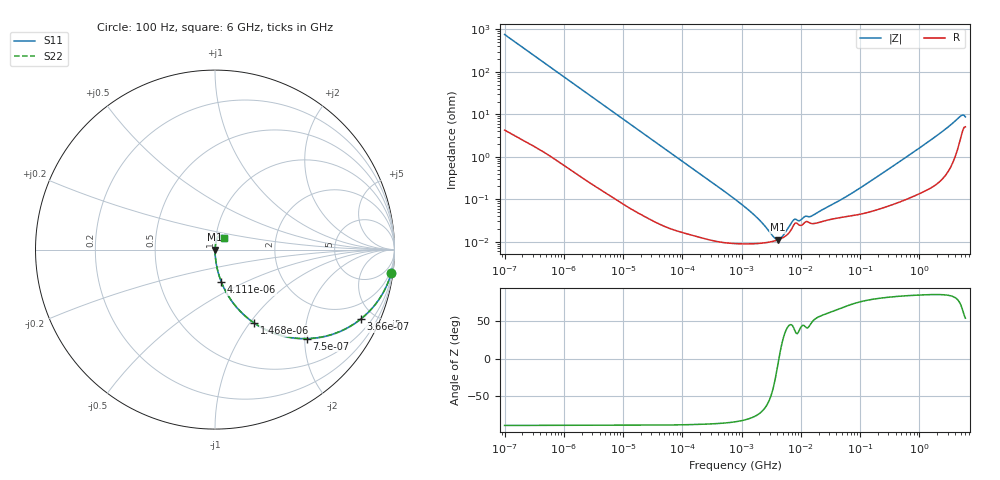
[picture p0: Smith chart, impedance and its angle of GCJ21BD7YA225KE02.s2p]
!Murata Part Number: GCJ21BD7YA225KE02
!These Parameters are Measured in Series Mode Connection
!Data Generated on Mar 13, 2026
!  o--ll--o
!Port1  Port2
!  o------o
!Operation Temp=25[degC], DC Bias Voltage=0[V]
!Freq. Start=100[Hz] Stop=6[GHz] 401[Steps]
# Hz S RI R 50
!Freq.(Hz) S11(Real) S11(Imag) S21(Real) S21(Imag) S12(Real) S12(Imag) S22(Real) S22(Imag)
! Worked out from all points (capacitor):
!   401 points, 100 Hz to 6 GHz, reference 50 ohm
!   read as one part in series: C = 2.09 uF near 109 Hz
!   lowest |Z| = 11.2 mohm at 4.06 MHz (marker M1)
!   series resonance near 4.274 MHz, so ESL is about 660 pH
!   S11 on the Smith chart (normalised r, x): 100 Hz: 1, -15; 366 Hz: 1.03, -4.16; 750 Hz: 1.02, -2.04; 1.468 kHz: 1.01, -1.05; 4.111 kHz: 1.00, -0.38; 6 GHz: 1.10, +0.14
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100  0.9822 -0.1294  0.0178 0.1294  0.0178 0.1294  0.9822 -0.1294
205  0.931 -0.2501  0.069 0.2501  0.069 0.2501  0.931 -0.2501
366  0.8107 -0.388  0.1893 0.388  0.1893 0.388  0.8107 -0.388
750  0.5103 -0.4959  0.4897 0.4959  0.4897 0.4959  0.5103 -0.4959
1468  0.217 -0.4081  0.783 0.4081  0.783 0.4081  0.217 -0.4081
2008  0.1302 -0.3323  0.8698 0.3323  0.8698 0.3323  0.1302 -0.3323
4111  0.0356 -0.1809  0.9644 0.1809  0.9644 0.1809  0.0356 -0.1809
10527  0.00613 -0.0733  0.9939 0.0733  0.9939 0.0733  0.00613 -0.0733
40335  0.000638 -0.0194  0.9994 0.0194  0.9994 0.0194  0.000638 -0.0194
774597  9.1e-05 -0.000996  0.9999 0.000996  0.9999 0.000996  9.1e-05 -0.000996
1734173  9.01e-05 -0.000385  0.9999 0.000385  0.9999 0.000385  9.01e-05 -0.000385
3549919  0.000104 -7.02e-05  0.9999 7.02e-05  0.9999 7.02e-05  0.000104 -7.02e-05
4060267  0.00011 -1.93e-05  0.9999 1.93e-05  0.9999 1.93e-05  0.00011 -1.93e-05
4856642  0.000122 4.91e-05  0.9999 -4.91e-05  0.9999 -4.91e-05  0.000122 4.91e-05
7599586  0.000247 0.000215  0.9998 -0.000215  0.9998 -0.000215  0.000247 0.000215
9506416  0.000245 0.000194  0.9998 -0.000194  0.9998 -0.000194  0.000245 0.000194
1.555665e7  0.000267 0.00031  0.9997 -0.00031  0.9997 -0.00031  0.000267 0.00031
6.518806e7  0.000399 0.0012  0.9996 -0.0012  0.9996 -0.0012  0.000399 0.0012
3.124326e8  0.000729 0.00523  0.9993 -0.00523  0.9993 -0.00523  0.000729 0.00523
1.873145e9  0.00304 0.0296  0.997 -0.0296  0.997 -0.0296  0.00304 0.0296
4.796499e9  0.0284 0.0799  0.9716 -0.0799  0.9716 -0.0799  0.0284 0.0799
6e9  0.0527 0.0636  0.9473 -0.0636  0.9473 -0.0636  0.0527 0.0636
